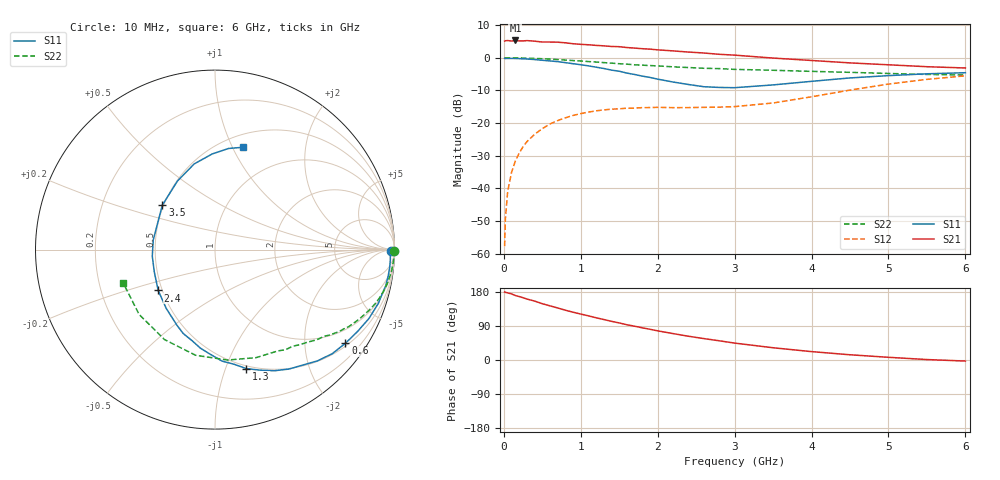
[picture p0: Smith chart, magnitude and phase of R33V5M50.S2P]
! SIEMENS Small Signal Semiconductors
! BFR181
! Si NPN RF Bipolar Junction Transistor in SOT23
! VCE = 3.5 V  IC = 0.5 mA
! Common Emitter S-Parameters:  May  1996
# GHz  S  MA  R  50
!  f  S11  S21  S12  S22
! GHz  MAG  ANG  MAG  ANG  MAG  ANG  MAG  ANG
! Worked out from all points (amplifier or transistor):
!   36 points, 10 MHz to 6 GHz, reference 50 ohm
!   highest |S21| = 5.3 dB at 150 MHz (marker M1)
!   |S21| within 3 dB of that: start of sweep to 2.075 GHz
!   unconditionally stable (mu >= 1): 2.372 GHz to 3.942 GHz
!   at 250 MHz: K = 0.12, MSG = 16.2 dB, |S12| = -27.2 dB
!   at 1.4 GHz: K = 0.61, MSG = 9.6 dB, |S12| = -15.8 dB
!   at 6 GHz: K = 0.92, MSG = 1.2 dB, |S12| = -5.5 dB
!   S11 on the Smith chart (normalised r, x): 10 MHz: 83, -35; 600 MHz: 0.57, -3.01; 1.3 GHz: 0.47, -1.18; 2.4 GHz: 0.48, -0.25; 3.5 GHz: 0.49, +0.29; 6 GHz: 0.63, +1.10
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0.01  0.9797 -0.5  1.802 179.7  0.0013 94.4  0.9994 -0.3
0.02  0.9753 -1.0  1.824 178.5  0.0034 89.6  0.9966 -0.6
0.05  0.9786 -3.0  1.836 177.2  0.009 88.5  0.9981 -1.4
0.1  0.9785 -5.7  1.807 174.4  0.0175 85.2  0.9971 -2.9
0.15  0.976 -8.9  1.843 170.1  0.0263 82.7  0.9952 -4.4
0.2  0.9719 -12.1  1.811 167.4  0.0347 82.0  0.993 -5.6
0.3  0.9585 -18.1  1.834 160.9  0.0519 77.7  0.9861 -8.5
0.4  0.9398 -24.1  1.798 155.5  0.0672 73.5  0.978 -11.3
0.6  0.8947 -35.7  1.743 142.9  0.0968 65.7  0.9546 -16.5
0.8  0.8425 -47.4  1.697 131.4  0.1204 58.3  0.9234 -21.4
1.1  0.7517 -63.9  1.582 116.5  0.1473 49.5  0.8756 -27.8
1.3  0.6854 -75.3  1.524 106.8  0.1592 44.3  0.8437 -31.5
1.5  0.6225 -86.4  1.479 97.8  0.1655 40.3  0.8115 -35.1
1.8  0.5238 -104.0  1.378 84.9  0.1723 36.4  0.7707 -39.4
2.2  0.4253 -129.8  1.275 69.7  0.1723 34.1  0.7268 -45.4
2.4  0.3898 -144.3  1.224 62.7  0.1726 34.3  0.7092 -48.4
3  0.3482 171.1  1.098 44.6  0.1787 40.6  0.6643 -58.2
3.5  0.3841 139.8  0.99 32.3  0.203 47.3  0.6439 -69.2
4.5  0.4914 103.6  0.835 13.8  0.3199 50.3  0.5985 -100.4
5  0.533 91.7  0.781 7.1  0.3955 45.0  0.5749 -119.3
5.5  0.5684 82.4  0.73 1.2  0.4671 37.5  0.5561 -139.5
6  0.5907 74.8  0.698 -2.8  0.5289 28.8  0.5439 -159.9
